PROGRAM MAIN
VAR
	dataout AT %Q* : BOOL;
	data_anolg AT %I* : INT;
	data_anolg_old : INT;
		
	ReadTimerModbus : TON;
	
	
	Master: ModbusRtuMasterV2_PcCOM;
	ReadErrorID : MODBUS_ERRORS;
	ReadBytes : UINT;
	WriteErrorID : MODBUS_ERRORS;
	
	ReadValue : INT;
	WriteValue: INT;
	
	ReadInput : INT;
	
	ExecuteRead : BOOL := FALSE;
	ExecuteWrite : BOOL := FALSE;
	
	
	
END_VAR


IF(_TaskInfo[GETCURTASKINDEXEX()].FirstCycle) THEN
	ReadTimerModbus(PT := T#100MS, IN := TRUE); //read every 100 ms from Modbus slaves
	data_anolg_old := data_anolg+150; //make sure to send first analog value to all Modbus slaves (Hystheresis)
END_IF

//Serve timer for Modbus read slaves
ReadTimerModbus();
ReadTimerModbus.IN := NOT ReadTimerModbus.Q;

//set output according to modbus slave discrete register value
dataout := INT_TO_BOOL(ReadInput);

//Execute modbus read
IF(ReadTimerModbus.Q) THEN
	ExecuteWrite := FALSE; //deactive write
	ExecuteRead := TRUE; //enable read
ELSE
	ExecuteRead := FALSE; //if timer not ellapsed - do no read
END_IF

//execute modbus write
IF ABS(data_anolg_old-data_anolg) > 20 THEN //only if analog value hystheresis of 50 digits exceeded
	ExecuteRead := FALSE; //deactivate read
	ExecuteWrite := TRUE; //enable write
	WriteValue := data_anolg_old; //set write value for modbus
	data_anolg_old := data_anolg; //remember new value
END_IF

// Set up MODBUS function blocks
// Modbus slave adress = 5
// Modbuss discrete register adress = 1 (see HMIDesigner project)
Master.ReadInputStatus(
	UnitID:= 5, 
	Quantity:= 1, 
	MBAddr:= 1, 
	cbLength:= 1, 
	pMemoryAddr:= ADR(ReadInput), 
	AuxQuantity:= , 
	AuxMBAddr:= , 
	AuxcbLength:= , 
	pAuxMemoryAddr:= , 
	Execute:= ExecuteRead, 
	Timeout:= T#10MS, 
	BUSY=> , 
	Error=> , 
	ErrorId=> ReadErrorID, 
	cbRead=> ReadBytes);

 // Modbus slave adress = 5
 // Modbuss holding register adress = 200 (see HMIDesigner project)
Master.WriteRegs(
	UnitID:= 5, 
	Quantity:= 1, 
	MBAddr:= 200, 
	cbLength:= SIZEOF(WriteValue), 
	pMemoryAddr:= ADR(WriteValue), 
	AuxQuantity:= , 
	AuxMBAddr:= , 
	AuxcbLength:= , 
	pAuxMemoryAddr:= , 
	Execute:= ExecuteWrite, 
	Timeout:= , 
	BUSY=> , 
	Error=> , 
	ErrorId=> WriteErrorID, 
	cbRead=> );

END_PROGRAM
